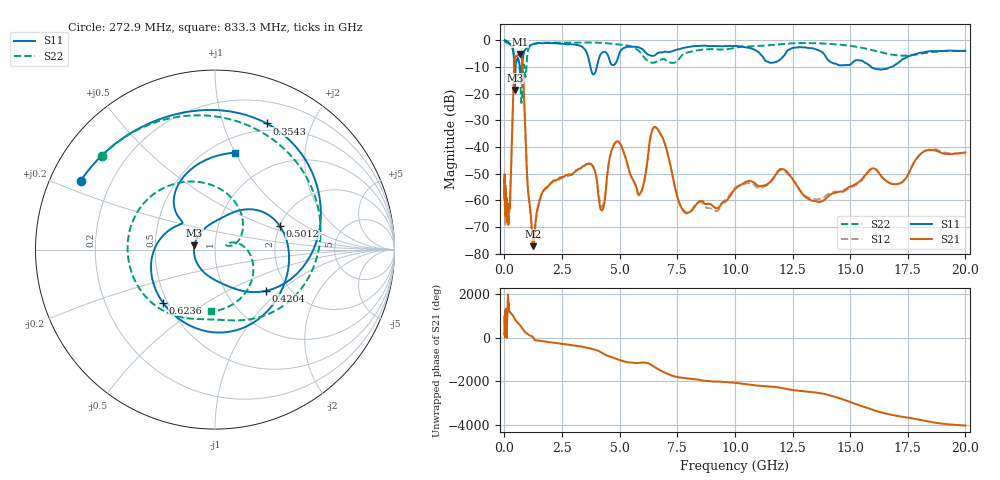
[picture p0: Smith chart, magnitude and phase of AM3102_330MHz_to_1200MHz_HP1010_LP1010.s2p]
! Date/Time: Tue, Sep 11, 2018 5:19 PM
! Network Analyzer: Agilent Technologies E8362B Rev: A.07.50.63
! Sweep from 0.010 to 20.000 GHz, 1601 Points, Sweep Type: LOG
! Power Supply: 4.949 V, 0.001 A
# Hz S DB R 50
!freq MagS11 AngS11 MagS21 AngS21 MagS12 AngS12 MagS22 AngS22
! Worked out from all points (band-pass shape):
!   1601 points, 10 MHz to 20 GHz, reference 50 ohm
!   highest |S21| = -5.13 dB at 676.1 MHz (marker M1); lowest = -77.2 dB at 1.242 GHz (marker M2)
!   |S21| within 3 dB of the highest: 435.5 MHz to 771.5 MHz (336 MHz wide, 55.7 % of centre)
!   lowest |S11| = -18.6 dB at 451.5 MHz (marker M3), VSWR 1.27, Z = 39.7 + j1.92 ohm
!   |S11| at or under -10 dB: 675.9 MHz to 768.8 MHz (92.86 MHz wide, 12.9 % of centre); 3.733 GHz to 4.006 GHz (273.2 MHz wide, 7.06 % of centre); 15.91 GHz to 16.77 GHz (859.8 MHz wide, 5.26 % of centre)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
!   |S22| runs from -23.4 to -0.2 dB; largest |S21 - S12| = 0.0099
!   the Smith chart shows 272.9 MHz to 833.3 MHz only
!   S11 on the Smith chart (normalised r, x): 272.9 MHz: 0.09, +0.24; 354.3 MHz: 0.42, +1.40; 420.4 MHz: 1.54, -0.82; 501.2 MHz: 2.01, +0.61; 623.6 MHz: 0.47, -0.34; 833.3 MHz: 0.64, +1.00
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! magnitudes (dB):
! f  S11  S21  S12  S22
! 10 MHz  0.0  -53.9  -51.5  -0.2
! 35.55 MHz  0.0  -63.0  -63.2  -0.4
! 126.4 MHz  -0.4  -63.0  -63.7  -0.9
! 272.9 MHz  -1.5  -52.6  -53.4  -1.7
! 354.3 MHz  -2.4  -28.7  -28.8  -3.2
! 420.4 MHz  -8.7  -10.5  -10.5  -6.6
! 447.2 MHz  -18.5  -7.0  -7.1  -8.1
! 451.5 MHz  -18.6  -6.7  -6.8  -8.2
! 501.2 MHz  -8.3  -5.8  -5.9  -6.7
! 623.6 MHz  -7.7  -5.2  -5.3  -8.1
! 676.1 MHz  -10.0  -5.1  -5.2  -12.3
! 743.5 MHz  -12.1  -6.3  -6.3  -23.4
! 833.3 MHz  -5.2  -17.0  -17.1  -9.2
! 1.242 GHz  -1.5  -77.2  -75.7  -1.3
! 1.59 GHz  -1.0  -58.2  -58.1  -0.9
! 3.668 GHz  -7.4  -46.3  -46.1  -0.8
! 4.23 GHz  -4.7  -63.8  -62.5  -0.9
! 4.902 GHz  -7.2  -37.9  -38.0  -1.5
! 5.652 GHz  -2.4  -53.5  -53.8  -2.9
! 6.58 GHz  -5.2  -32.7  -32.8  -8.0
! 7.92 GHz  -2.5  -64.9  -64.6  -4.6
! 20 GHz  -3.9  -42.0  -42.5  -3.9
